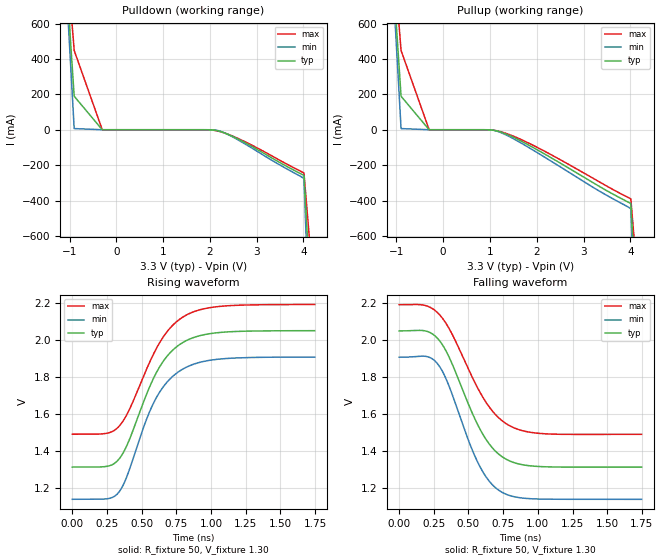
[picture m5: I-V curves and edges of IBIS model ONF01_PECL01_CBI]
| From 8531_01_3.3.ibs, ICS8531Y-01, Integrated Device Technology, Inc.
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[Model]   ONF01_PECL01_CBI
Model_type   Output_ECL
Polarity   Non-Inverting
|   typ   min   max
C_comp   2pF   1.5pF   2.5pF
Vmeas = 1.645V
Rref = 50
Cref = 0
Vref = 1.3V
|   typ   min   max
[Voltage range]   3.3V   3.135V   3.465V
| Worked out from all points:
|   rising waveform, R_fixture 50, V_fixture 1.30: 20-80 % time 262ps typ, 254ps min, 274ps max; typ from 1.31 V to 2.05 V
|   falling waveform, R_fixture 50, V_fixture 1.30: 20-80 % time 265ps typ, 241ps min, 289ps max; typ from 2.05 V to 1.31 V
[Pulldown]
|Voltage   I (typ)   I (min)   I (max)
-3.3V     9.786A     12.03A     8.45A
-1.5V     2.58A      2.839A     2.441A
-900mV    189.2mA    6.554mA    448mA
-300mV    38.6nA     137.1pA    1.11uA
1.929V    -65.47uA   -9.735uA   -208.8uA
2.126V    -3.6mA     -2.093mA   -4.912mA
2.225V    -10.1mA    -8.738mA   -11.16mA
2.422V    -30.08mA   -31.69mA   -29.07mA
2.767V    -75.59mA   -82.9mA    -70mA
4.01V     -258.5mA   -276.6mA   -244.2mA
4.528V    -2.686A    -3.931A    -1.893A
6.6V      -15.7A     -20.54A    -12.73A
[Pullup]
|Voltage   I (typ)   I (min)   I (max)
-3.3V     9.786A     12.03A     8.45A
-1.5V     2.58A      2.839A     2.441A
-900mV    189.2mA    6.554mA    448mA
-300mV    38.6nA     137.1pA    1.11uA
1.041V    -1.672mA   -1.458mA   -1.662mA
1.288V    -18.76mA   -22.48mA   -15.85mA
1.682V    -66.53mA   -77.82mA   -57.33mA
2.274V    -153.4mA   -172.3mA   -136.6mA
3.26V     -308.2mA   -334.6mA   -282.9mA
4.01V     -417.2mA   -447.3mA   -390.5mA
4.528V    -2.844A    -4.101A    -2.04A
6.6V      -15.79A    -20.6A     -12.84A
[Ramp]
|   typ   min   max
dV/dt_r   0.59/0.411n   0.615/0.404n   0.561/0.427n
dV/dt_f   0.592/0.403n   0.62/0.365n   0.562/0.44n
R_load =   50.0000
[Rising Waveform]
R_fixture = 50
V_fixture = 1.30   | VCC_typ - 2V
V_fixture_max = 1.465   | VCC_max - 2V
V_fixture_min = 1.135   | VCC_min - 2V
C_fixture = 0.0p
| Time   typ   min   max
0s        1.314V     1.139V     1.491V
247ps     1.317V     1.141V     1.496V
332.8ps   1.353V     1.175V     1.531V
409.9ps   1.458V     1.295V     1.622V
522ps     1.682V     1.545V     1.819V
595.6ps   1.809V     1.674V     1.94V
686.7ps   1.916V     1.776V     2.049V
793.5ps   1.986V     1.842V     2.123V
1.063ns   2.041V     1.898V     2.183V
1.748ns   2.051V     1.908V     2.193V
[Falling Waveform]
R_fixture = 50
V_fixture = 1.30   | VCC_typ - 2V
V_fixture_max = 1.465   | VCC_max - 2V
V_fixture_min = 1.135   | VCC_min - 2V
C_fixture = 0.0p
| Time   typ   min   max
0s        2.051V     1.909V     2.193V
197.9ps   2.049V     1.912V     2.187V
282ps     2.006V     1.868V     2.146V
364.4ps   1.902V     1.743V     2.058V
571.1ps   1.536V     1.333V     1.735V
649.9ps   1.438V     1.237V     1.639V
735.7ps   1.373V     1.18V      1.569V
846.1ps   1.334V     1.151V     1.521V
995ps     1.317V     1.141V     1.497V
1.748ns   1.314V     1.139V     1.491V
